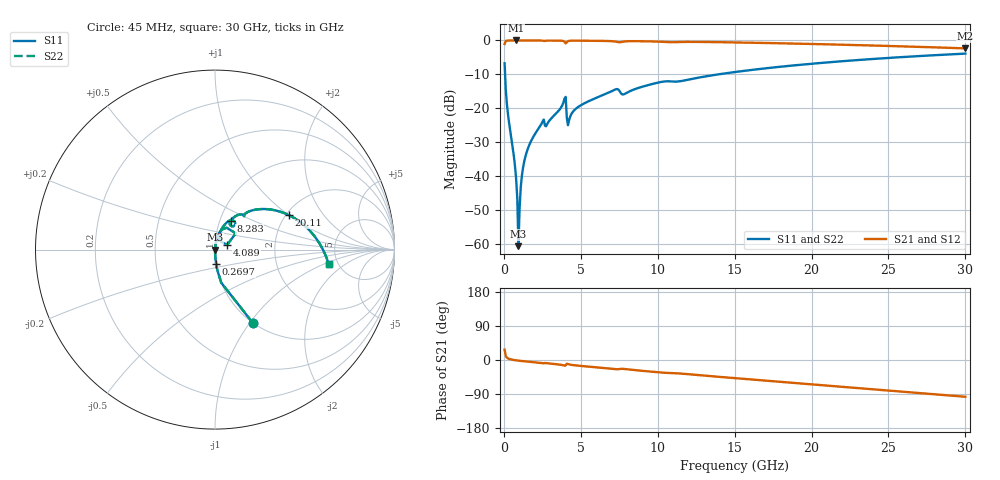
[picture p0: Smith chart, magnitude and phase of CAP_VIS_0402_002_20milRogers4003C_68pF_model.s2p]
! S-parameter model data by Modelithics Inc.  support@modelithics.com  813-866-6335  Tampa FL USA
! S-Parameter data specifications:
! Substrate: 20-mil Rogers 4003C, substrate thickness, H=0.508mm, Dielectric constant, Er=3.75
! PCB Mounting Pad Footprint: Pad width, PadW=0.50mm , Pad length, PadL=0.50mm , Pad gap, PadG (edge-to-edge)=0.40mm , Reference planes=1.4mm apart
! Created Wed Nov 18 12:56:31 2015
# hz S ma R 50
! 2 Port Network Data from SP1.SP block
! freq  magS11  angS11  magS21  angS21  magS12  angS12  magS22  angS22
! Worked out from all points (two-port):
!   401 points, 45 MHz to 30 GHz, reference 50 ohm
!   highest |S21| = -0.01 dB at 793.9 MHz (marker M1); lowest = -2.3 dB at 30 GHz (marker M2)
!   |S21| within 3 dB of the highest: start of sweep to end of sweep
!   lowest |S11| = -60.7 dB at 943.6 MHz (marker M3), VSWR 1.00, Z = 50.1 - j0.0567 ohm
!   |S11| at or under -10 dB: 76.32 MHz to 13.96 GHz (13.88 GHz wide, 198 % of centre)
!   |S22| runs from -60.7 to -3.9 dB; largest |S21 - S12| = 0
!   S11 on the Smith chart (normalised r, x): 45 MHz: 1.00, -1.03; 269.7 MHz: 1.00, -0.16; 4.089 GHz: 1.14, +0.06; 8.283 GHz: 1.12, +0.37; 20.11 GHz: 2.08, +1.00; 30 GHz: 4.20, -1.17
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4.5e7  0.4594 -62.7  0.888 27.3  0.888 27.3  0.4594 -62.7
2.696625e8  0.07936 -85.6  0.9964 4.1  0.9964 4.1  0.07936 -85.6
6.441e8  0.01976 -88.3  0.9992 -0.1  0.9992 -0.1  0.01976 -88.3
7.93875e8  0.009096 -86.6  0.9992 -1.0  0.9992 -1.0  0.009096 -86.6
9.4365e8  0.0009201 -38.0  0.9992 -1.7  0.9992 -1.7  0.0009201 -38.0
1.093425e9  0.006772 80.8  0.9991 -2.4  0.9991 -2.4  0.006772 80.8
1.168312e9  0.01008 82.6  0.9991 -2.7  0.9991 -2.7  0.01008 82.6
1.318088e9  0.01626 83.5  0.999 -3.4  0.999 -3.4  0.01626 83.5
1.8423e9  0.03545 82.8  0.9982 -5.4  0.9982 -5.4  0.03545 82.8
2.4414e9  0.05878 79.4  0.9954 -7.9  0.9954 -7.9  0.05878 79.4
3.864262e9  0.1208 69.7  0.9796 -14.1  0.9796 -14.1  0.1208 69.7
4.088925e9  0.07267 21.1  0.9368 -9.7  0.9368 -9.7  0.07267 21.1
4.2387e9  0.06687 68.4  0.9862 -11.6  0.9862 -11.6  0.06687 68.4
5.062462e9  0.1126 72.9  0.9911 -15.8  0.9911 -15.8  0.1126 72.9
7.2342e9  0.1886 60.4  0.9642 -24.2  0.9642 -24.2  0.1886 60.4
8.282625e9  0.1824 61.7  0.9751 -25.8  0.9751 -25.8  0.1824 61.7
1.007992e10  0.2403 54.7  0.9589 -32.6  0.9589 -32.6  0.2403 54.7
1.50225e10  0.342 41.3  0.9346 -47.9  0.9346 -47.9  0.342 41.3
2.003996e10  0.4535 25.1  0.8866 -64.4  0.8866 -64.4  0.4535 25.1
2.011485e10  0.4551 24.9  0.8858 -64.6  0.8858 -64.6  0.4551 24.9
2.505742e10  0.5529 8.8  0.8282 -80.8  0.8282 -80.8  0.5529 8.8
3e10  0.6391 -7.4  0.7635 -97.0  0.7635 -97.0  0.6391 -7.4
